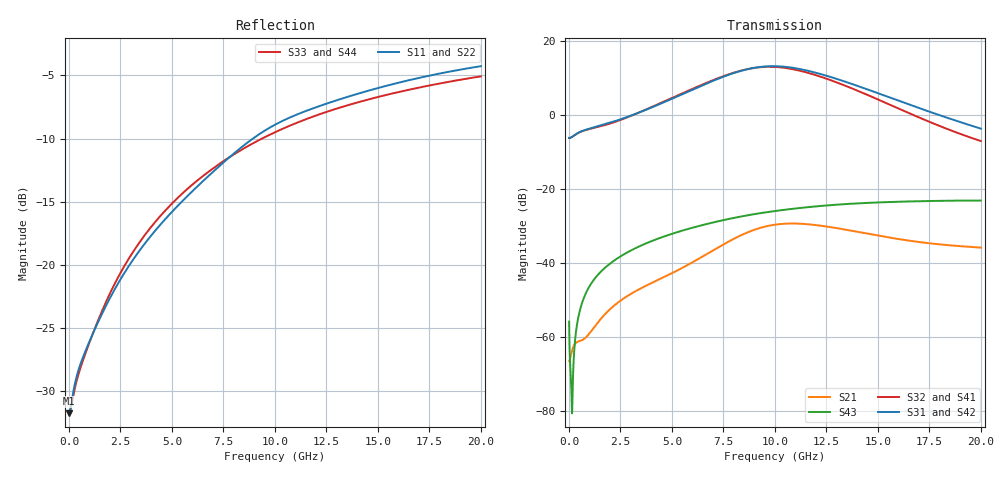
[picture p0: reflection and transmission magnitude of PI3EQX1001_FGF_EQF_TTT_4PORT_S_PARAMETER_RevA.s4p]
! NPort=4 DATA=2000 NOISE=0 GROUPDELAY=0 COMPLEX_DATAFORMAT=POLAR
! NumOfBlock=1 NumOfParam=0
! .MODEL Smodel S TSTONEFILE=PI3EQX1001_FGF_EQF_TTT_4PORT_S_PARAMETER_RevA.s4p TYPE=S
!  -- The above .MODEL line can be used for the S element in the netlist.
! The s parameter is extracted from the linear redriver, it is not bi-directional; only s(4,1)s(4,2) and s(3,1)s(3,2)
! should be the insertion loss
!Port definition:
!Port1 = input+
!Port2 = input¨C
!Port3 = output+
!Port4 = output-
# Hz S MA R  50
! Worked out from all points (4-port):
!   2000 points, 10 MHz to 20 GHz, reference 50 ohm
!   strongest paths, dB at 10 MHz, 5.01 GHz, 10.01 GHz, 15.01 GHz, 20 GHz:
!     S31: -6.1, 4.5, 13.3, 6.0, -3.6
!     S42: -6.1, 4.5, 13.3, 6.0, -3.6
!     S32: -6.1, 4.7, 13.1, 4.3, -6.9
!     S41: -6.1, 4.7, 13.1, 4.2, -7.0
!     S43: -55.8, -32.0, -25.9, -23.5, -23.0
!     S21: -66.4, -42.7, -29.6, -32.5, -35.8
!   lowest |S11| = -31.7 dB at 10 MHz (marker M1), VSWR 1.05, Z = 47.5 - j0.063 ohm
!   |S11| at or under -10 dB: start of sweep to 8.929 GHz
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1e7  0.02591 -178.5  0.0004922 2.7  3.669e-05 -0.2  4.787e-05 -0.1
     0.0004763 2.9  0.02597 -178.7  4.577e-05 -0.2  5.994e-05 -0.1
     0.496 -0.1  0.496 179.9  0.02616 178.4  0.001615 -59.2
     0.4957 179.9  0.4958 -0.1  0.001626 -58.9  0.02612 178.4
6.88e9  0.2291 -105.3  0.0136 89.8  2.208e-05 -30.9  3.226e-05 -29.6
        0.01428 88.1  0.2273 -105.3  2.92e-05 -25.9  4.045e-05 -24.8
        2.844 -54.5  2.909 129.7  0.2372 -111.7  0.03502 57.0
        2.899 129.7  2.839 -54.4  0.03499 57.1  0.2372 -111.7
8.89e9  0.3146 -107.6  0.0266 64.9  1.989e-05 -27.8  3.25e-05 -32.6
        0.02763 63.4  0.3125 -107.6  3.014e-05 -25.9  3.827e-05 -24.1
        4.348 -112.1  4.34 72.0  0.3016 -114.4  0.04569 44.6
        4.321 72.1  4.344 -112.0  0.04564 44.5  0.3015 -114.3
1.066e10  0.3812 -112.7  0.03326 30.5  2.195e-05 -21.9  3.363e-05 -42.7
          0.03445 29.3  0.3784 -112.8  3.182e-05 -35.2  4.027e-05 -22.8
          4.49 -172.4  4.321 12.1  0.354 -117.2  0.05383 32.9
          4.3 12.3  4.486 -172.3  0.05371 32.9  0.3538 -117.2
1.307e10  0.4503 -118.3  0.02859 -4.3  2.897e-05 -36.8  3.008e-05 -63.7
          0.02965 -5.4  0.4466 -118.3  2.836e-05 -54.3  4.648e-05 -33.9
          3.074 116.8  2.748 -57.3  0.4175 -121.3  0.06233 17.1
          2.733 -57.0  3.071 116.9  0.0622 17.1  0.4174 -121.2
1.564e10  0.5174 -123.0  0.02118 -21.3  2.873e-05 -69.4  2.201e-05 -92.4
          0.02207 -22.4  0.5131 -123.0  1.987e-05 -79.0  4.35e-05 -56.5
          1.72 59.6  1.372 -110.5  0.4758 -125.2  0.06754 1.1
          1.364 -110.0  1.718 59.7  0.06748 1.2  0.4754 -125.2
2e10  0.6119 -130.6  0.01566 -27.2  1.512e-05 -149.3  1.249e-05 148.3
      0.0163 -29.2  0.6065 -130.6  8.062e-06 131.9  1.789e-05 -96.1
      0.6617 -10.0  0.4498 -161.7  0.5577 -131.1  0.07056 -23.4
      0.4486 -160.8  0.6606 -9.9  0.07053 -23.4  0.5576 -131.1
